PROGRAM MAIN
VAR CONSTANT	
    cInitSource			: ST_MA_MultiArray_InitPars := ( eTypeCode := eMA_TypeCode_LREAL, nDims := 1, aDimSizes := [cBufferLength]);	
END_VAR
VAR
	(* input selection *)
	nInputSelection				: UDINT := 1;						// Switch between hardware and function generator	
	nSample						: UDINT;
	aEl3632 AT %I*				: ARRAY[1..cOversamples] OF INT;	// Input from hardware e.g. EL3632
	
	(* signal generation *)
	fbFunctionGenerator_Carrier		: FB_FunctionGenerator;
	fbFunctionGenerator_Fault		: FB_FunctionGenerator;
	fbFunctionGenerator_Shock		: FB_FunctionGenerator;
	fbFunctionGenerator_Shockwave	: FB_FunctionGenerator;							
	
	(* signal parts *)
	aBufferCarrier				: ARRAY [1..cOversamples] OF LREAL;
	aBufferShockwave			: ARRAY [1..cOversamples] OF LREAL;
	aBuffer						: ARRAY [1..cOversamples] OF LREAL;
	
	(* Source and Sink of analysis chain *)
	fbSource					: FB_CMA_Source :=(	stInitPars := cInitSource, nOwnID := eID_Source, aDestIDs := [eID_SESpectrum]);	// Initialize source buffers
	fbSink						: FB_CMA_Sink 	:= (nOwnID := eID_Sink);
	
	(* SpikeEnergy spectrum result *)
	aSESpectrumResult		: ARRAY[1..cFFTResult] OF LREAL;	// Copy of result
	
	i : UDINT;
END_VAR

CASE nInputSelection OF
	0:  (* input from EL3632 *)
		FOR nSample := 1 TO cOversamples DO
			aBuffer[nSample] := INT_TO_LREAL(aEl3632[nSample]);
		END_FOR
	1:  (* signal generator *)		
		GenerateSignal();
END_CASE	

(* Call source to collect data. *)
fbSource.Input1DStd( pDataIn 		:= ADR(aBuffer),
				  	nDataInSize 	:= SIZEOF(aBuffer), 
				  	eElementType 	:= eMA_TypeCode_LREAL,
				  	nOptionPars		:= cCMA_Option_MarkInterruption ); 
IF fbSource.bError THEN
	fbErrHist.AddError(bErr:=TRUE, hrErrCode:=fbSource.hrErrorCode, sErrSource:='MAIN.fbSource'); // error monitoring
	// ToDo: if error
END_IF

(* Push results to sink *)
fbSink.Output1DStd(	pDataOut 		:= ADR(aSESpectrumResult), 
					nDataOutSize 	:= SIZEOF(aSESpectrumResult), 
					eElementType 	:= eMA_TypeCode_LREAL, 
					nOptionPars		:= 0);
IF fbSink.bError THEN
	fbErrHist.AddError(bErr:=TRUE, hrErrCode:=fbSink.hrErrorCode, sErrSource:='MAIN.fbSink'); // error monitoring
	// ToDo: if error
END_IF

METHOD GenerateSignal : BOOL
VAR_INPUT
END_VAR
VAR
	denum : LREAL;
END_VAR
fbFunctionGenerator_Carrier(	fFrequency 	:= cCarrierFrequency,
								fAmplitude 	:= cCarrierAmplitude,
								eFunction 	:= E_FunctionType.Sine,
								aSignal		:= aBufferCarrier,
								fSampleRate := cSampleRate);
								
fbFunctionGenerator_Shockwave(	fCarrierFrequency 	:= cDefectFrequency,
								fCarrierAmplitude 	:= cDefectAmplitude,
								fFrequency 			:= cShockFrequency,
								fAmplitude 			:= cShockAmplitude,
								eFunction 			:= E_FunctionType.Shockwave,
								nDutyCycle			:= cDefectDutyCycle,
								aSignal				:= aBufferShockwave,
								fSampleRate 		:= cSampleRate);

FOR i := 1 TO cOversamples DO
	denum := cCarrierAmplitude;
	IF denum > 0.0 THEN
		aBuffer[i] := aBufferCarrier[i] * (1.0 + (cDefectAmplitude / denum) * aBufferShockwave[i]);
	ELSE
		aBuffer[i] := aBufferShockwave[i];
	END_IF
END_FOR
END_METHOD

END_PROGRAM
